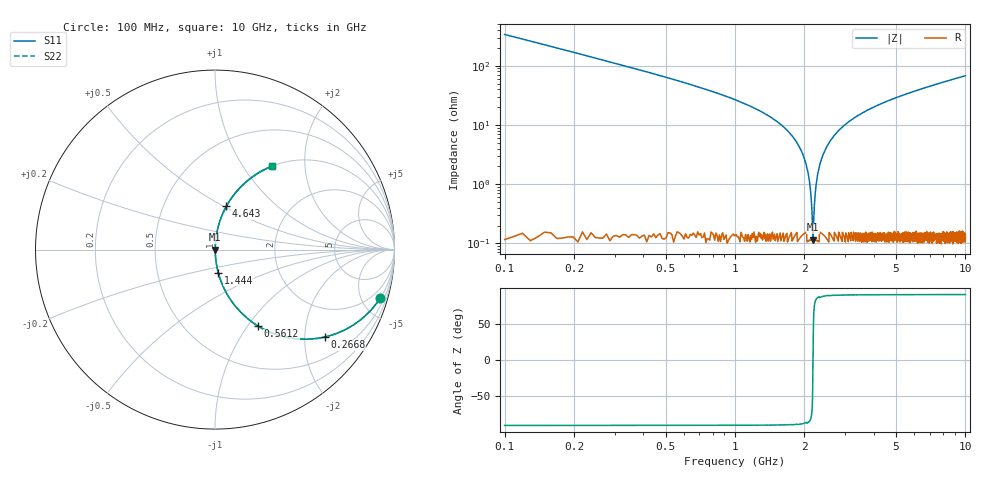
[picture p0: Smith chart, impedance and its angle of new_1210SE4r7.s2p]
!	AVX	Thin	Film	Operation	Date:	April 2007
!	Description:	Accu-P®	"Series,"	Thin	"Film,"	"SMD,"	RF	Capacitor
!	Part	Number:	12101J4R7ABT
!	100	MHz	-	5.05	GHz
!	Serial	Measurements
#	MHZ	S	MA	R	50
!	S11	S21	S12	S22
!	dB	Phase	dB	Phase	dB	Phase	dB	Phase
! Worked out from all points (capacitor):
!   1010 points, 100 MHz to 10 GHz, reference 50 ohm
!   read as one part in series: C = 4.7 pF near 149.1 MHz
!   lowest |Z| = 115 mohm at 2.18 GHz (marker M1)
!   series resonance near 2.181 GHz, so ESL is about 1.1 nH
!   S11 on the Smith chart (normalised r, x): 100 MHz: 1.00, -6.76; 266.8 MHz: 1.00, -2.50; 561.1 MHz: 1.00, -1.13; 1.444 GHz: 1.00, -0.26; 4.643 GHz: 1.00, +0.51; 10 GHz: 1.00, +1.36
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100  0.959 -16.5  0.284 73.5  0.284 73.5  0.959 -16.5
266.799  0.781 -38.6  0.624 51.3  0.624 51.3  0.781 -38.6
561.15  0.49 -60.5  0.87 29.4  0.87 29.4  0.49 -60.5
894.747  0.3 -72.3  0.953 17.4  0.953 17.4  0.3 -72.3
1444.202  0.13 -81.9  0.99 7.5  0.99 7.5  0.13 -81.9
1758.176  0.067 -85.0  0.996 3.9  0.996 3.9  0.067 -85.0
1924.975  0.039 -85.9  0.998 2.2  0.998 2.2  0.039 -85.9
2023.092  0.023 -85.5  0.998 1.3  0.998 1.3  0.023 -85.5
2081.962  0.014 -84.0  0.999 0.8  0.999 0.8  0.014 -84.0
2150.644  0.00451 -73.0  0.999 0.2  0.999 0.2  0.00451 -73.0
2180.079  0.0013 -4.6  0.999 0.0  0.999 0.0  0.0013 -4.6
2209.514  0.00426 72.0  0.999 -0.2  0.999 -0.2  0.00426 72.0
2258.573  0.011 82.6  0.999 -0.6  0.999 -0.6  0.011 82.6
2307.631  0.018 84.8  0.999 -1.0  0.999 -1.0  0.018 84.8
2494.054  0.042 85.8  0.998 -2.4  0.998 -2.4  0.042 85.8
2847.275  0.083 84.3  0.995 -4.8  0.995 -4.8  0.083 84.3
3406.541  0.142 81.3  0.989 -8.1  0.989 -8.1  0.142 81.3
4642.815  0.249 75.3  0.967 -14.4  0.967 -14.4  0.249 75.3
5054.906  0.281 73.4  0.959 -16.3  0.959 -16.3  0.281 73.4
6703.271  0.392 66.7  0.919 -23.1  0.919 -23.1  0.392 66.7
8351.635  0.484 60.9  0.874 -29.0  0.874 -29.0  0.484 60.9
10000  0.561 55.8  0.827 -34.1  0.827 -34.1  0.561 55.8
